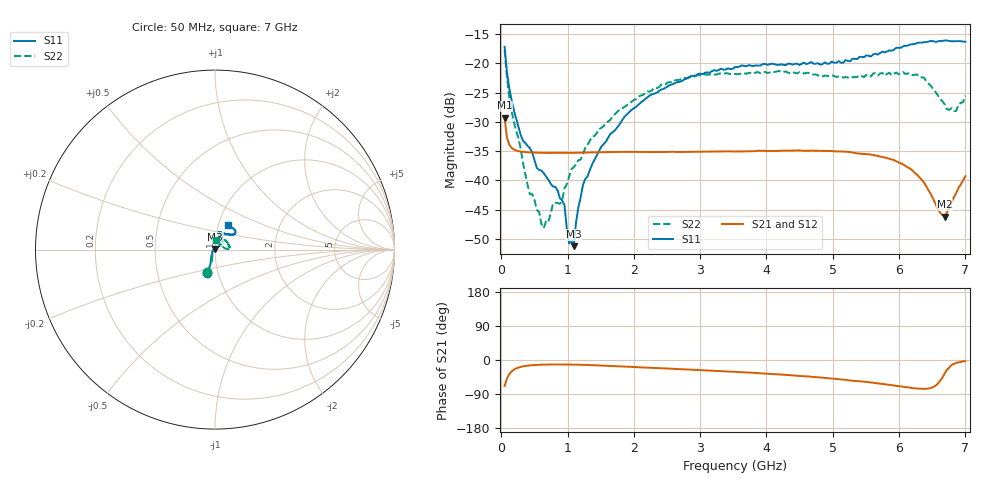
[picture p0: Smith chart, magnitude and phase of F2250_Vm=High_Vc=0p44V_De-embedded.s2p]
! Integrated Device Technology
! Corporate Headquarters
! 6024 Silver Creek Valley Road
! San Jose, CA 95138  USA
! Phone:  1-408-284-8200
! Toll Free:  1-800-223-1366
! Webpage:  http://www.idt.com/
! Timing and RF Division
! 515 Groton Road, Suite 102
! Westford, MA 01886-6024
! Device:  F2250
! Description: Voltage Variable RF Attenuator
! Frequency:  50.0 -  6000.00 MHz
! Package:  3x3 mm Thin QFN Plastic Package: 16 pin
! Ports:  2 RF, 3 DC
!  Pin  1  = GND
!  Pin  2  = NC
!  Pin  3  = RF1  = Port 1
!  Pin  4  = NC
!  Pin  5  = GND
!  Pin  6  = GND
!  Pin  7  = GND
!  Pin  8  = GND
!  Pin  9  = NC
!  Pin 10  = RF2  = Port 2
!  Pin 11  = NC
!  Pin 12  = GND
!  Pin 13  = GND
!  Pin 14  = VCNTRL
!  Pin 15  = VDD
!  Pin 16  = VMODE
! Vcntrl:  0.440 Volts
! Vmode:  +3.300 Volts
! Vdd:  +3.30  Volts
! Current:  1.264 mA
! Data:  The device was measured on a the F2250 evaluation board which has
!  individual transmission lines to the RF pins.  Data was collected
!  using a calibrated network analyzer.  The evaluation board was
!  de-embedded using a TRL calibration technique.
!  The reference plane is the edge of the package pin.
! Misc:  SN 10
!  Action Tracker AT0258
! Date Measured:  2014-11-26
! Date:  2015-10-15  MJV
! Note:
!  Integrated Device Technology supplies this data as a sample of measured
!  data at the package pin for this product.  Your particular data for this
!  product may vary.
!  Data was taken at 25 degrees C.
!  Integrated Device Technology reserves the right to change this data at anytime.
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# GHz S dB R 50
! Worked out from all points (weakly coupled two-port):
!   201 points, 50 MHz to 7 GHz, reference 50 ohm
!   highest |S21| = -29.29 dB at 50 MHz (marker M1); lowest = -46.2 dB at 6.687 GHz (marker M2)
!   lowest |S11| = -51.3 dB at 1.093 GHz (marker M3), VSWR 1.01, Z = 50 + j0.274 ohm
!   |S11| at or under -10 dB: start of sweep to end of sweep
!   |S22| runs from -48.2 to -17.7 dB; largest |S21 - S12| = 4.8e-05
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0.05  -17.17 -108.5  -29.29 -68.4  -29.29 -68.4  -17.73 -108.8
0.1195  -24.20 -112.0  -33.89 -37.5  -33.90 -37.5  -25.70 -107.7
0.29325  -32.27 -127.4  -35.09 -18.2  -35.09 -18.2  -34.62 -115.8
0.43225  -34.54 -145.3  -35.24 -14.2  -35.24 -14.2  -42.39 -150.7
0.5365  -37.90 -154.7  -35.29 -12.9  -35.29 -12.9  -45.06 -170.9
0.64075  -38.78 -162.5  -35.31 -12.2  -35.31 -12.2  -48.17 139.2
0.77975  -41.07 176.3  -35.32 -11.9  -35.33 -11.9  -43.95 107.2
0.91875  -43.45 156.0  -35.33 -11.9  -35.34 -11.9  -43.44 82.7
0.9535  -44.30 170.9  -35.33 -11.9  -35.33 -11.9  -41.35 87.5
1.023  -50.81 140.9  -35.32 -12.0  -35.32 -12.0  -39.38 70.8
1.0925  -51.26 89.9  -35.31 -12.2  -35.31 -12.2  -37.76 65.8
1.12725  -47.20 61.0  -35.30 -12.3  -35.30 -12.3  -37.27 59.1
1.2315  -40.82 40.6  -35.27 -12.7  -35.26 -12.7  -35.60 49.3
1.6485  -32.03 41.1  -35.18 -15.5  -35.18 -15.5  -29.62 46.4
2.37825  -24.75 46.6  -35.15 -21.5  -35.15 -21.5  -24.08 46.8
3.525  -20.66 71.7  -35.08 -31.3  -35.08 -31.3  -21.82 69.2
4.7065  -20.06 72.0  -34.94 -44.7  -34.94 -44.7  -21.92 68.2
5.85325  -17.79 40.5  -36.33 -65.5  -36.34 -65.6  -21.63 19.8
6.3745  -16.40 40.9  -40.37 -76.2  -40.40 -76.3  -22.43 3.5
6.68725  -16.12 47.8  -46.19 -35.6  -46.16 -35.3  -27.01 25.4
6.861  -16.22 54.5  -42.18 -7.7  -42.14 -7.6  -28.14 58.2
7  -16.33 62.4  -39.30 -3.3  -39.26 -3.4  -25.55 86.8
